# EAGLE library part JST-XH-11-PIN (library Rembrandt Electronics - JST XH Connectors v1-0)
JST XH Connector 2 Pin Wire to board connector. Pitch: 2,54 mm, (0.100") Number of pins: 11 Created by Rembrandt Electronics www.rembrandtelectronics.com
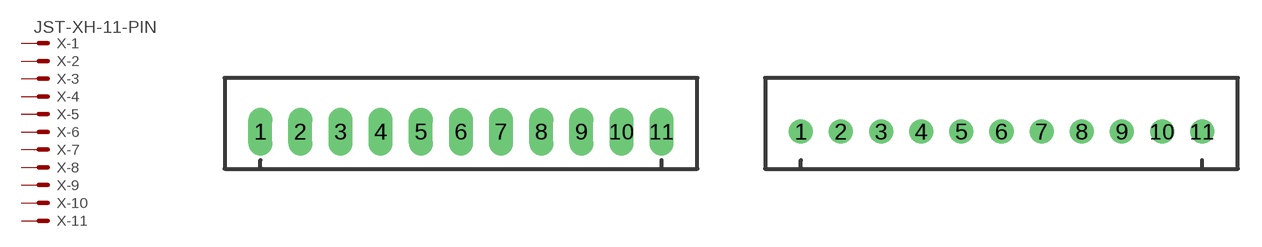
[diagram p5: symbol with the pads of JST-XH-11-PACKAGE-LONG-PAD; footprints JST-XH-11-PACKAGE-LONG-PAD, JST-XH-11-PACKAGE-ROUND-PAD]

Designator prefix X; gates -1=MV -2=M -3=M -4=M -5=M -6=M -7=M -8=M -9=M -10=M -11=M

## JST-XH-11-PIN-LONG-PAD  [JST-XH-11-PACKAGE-LONG-PAD]
1  -1:S  pas
2  -2:S  pas
3  -3:S  pas
4  -4:S  pas
5  -5:S  pas
6  -6:S  pas
7  -7:S  pas
8  -8:S  pas
9  -9:S  pas
10  -10:S  pas
11  -11:S  pas

## JST-XH-11-PIN-ROUND-PAD  [JST-XH-11-PACKAGE-ROUND-PAD]
Pads as for JST-XH-11-PACKAGE-LONG-PAD

## Footprint JST-XH-11-PACKAGE-LONG-PAD (pad centres in mm)
JST XH Connector Long Pads (Package) Wire to board connector. Pitch: 2,54 mm, (0.100") Number of pins: 11 Created by Rembrandt Electronics www.rembrandtelectronics.com
drill 1.016 long: 1 -12.7,0; 2 -10.16,0; 3 -7.62,0; 4 -5.08,0; 5 -2.54,0; 6 0,0; 7 2.54,0; 8 5.08,0; 9 7.62,0; 10 10.16,0; 11 12.7,0

## Footprint JST-XH-11-PACKAGE-ROUND-PAD (pad centres in mm)
JST XH Connector Round Pads (Package) Wire to board connector. Pitch: 2,54 mm, (0.100") Number of pins: 11 Created by Rembrandt Electronics www.rembrandtelectronics.com
drill 1.016: 1 -12.7,0; 2 -10.16,0; 3 -7.62,0; 4 -5.08,0; 5 -2.54,0; 6 0,0; 7 2.54,0; 8 5.08,0; 9 7.62,0; 10 10.16,0; 11 12.7,0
